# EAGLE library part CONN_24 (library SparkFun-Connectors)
Multi connection point. Often used as Generic Header-pin footprint for 0.1 inch spaced/style header connections On any of the 0.1 inch spaced packages, you can populate with these: Break Away Headers - Straight (PRT-00116) Break Away Male Headers - Right Angle (PRT-00553) Female Headers (PRT-00115) Break Away Headers - Machine Pin (PRT-00117) Break Away Female Headers - Swiss Machine Pin (PRT-00743) For SCREWTERMINALS and SPRING TERMINALS visit here: Screw Terimnals on SparkFun.com (5mm/3.5mm/2.54mm spacing) This device is also useful as a general connection point to wire up your design to another part of your project. Our various solder wires solder well into these plated through hole pads. Hook-Up Wire - Assortment (Stranded, 22 AWG) (PRT-11375) Hook-Up Wire - Assortment (Solid Core, 22 AWG) (PRT-11367) View the entire wire category on our website here Special notes: Molex polarized connector foot print use with SKU : PRT-08231 with associated crimp pins and housings. 1MM SMD Version SKU: PRT-10208 NOTES ON THE VARIANTS LOCK and LOCK_LONGPADS... This footprint was designed to help hold the alignment of a through-hole component (i.e. 6-pin header) while soldering it into place. You may notice that each hole has been shifted either up or down by 0.005 of an inch from it's more standard position (which is a perfectly straight line). This slight alteration caused the pins (the squares in the middle) to touch the edges of the holes. Because they are alternating, it causes a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
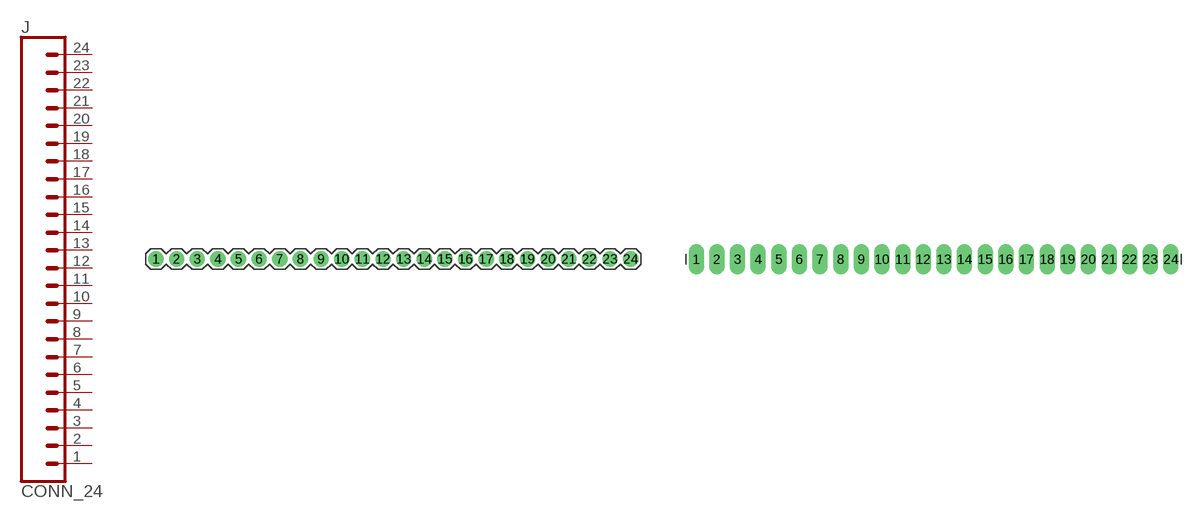
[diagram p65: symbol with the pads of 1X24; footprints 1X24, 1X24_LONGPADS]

Designator prefix J

## CONN_24  [1X24]
1  1  pas
2  2  pas
3  3  pas
4  4  pas
5  5  pas
6  6  pas
7  7  pas
8  8  pas
9  9  pas
10  10  pas
11  11  pas
12  12  pas
13  13  pas
14  14  pas
15  15  pas
16  16  pas
17  17  pas
18  18  pas
19  19  pas
20  20  pas
21  21  pas
22  22  pas
23  23  pas
24  24  pas

## CONN_24LONGPADS  [1X24_LONGPADS]
Pads as for 1X24

## CONN_24LOCK  [1X24_LOCK]
Pads as for 1X24

## Footprint 1X24 (pad centres in mm)
Plated Through Hole -24 Pin Specifications: Pin count:24 Pin pitch:0.1" Example device(s): CONN_24
drill 1.016 pad 1.88: 1 -26.67,0; 2 -24.13,0; 3 -21.59,0; 4 -19.05,0; 5 -16.51,0; 6 -13.97,0; 7 -11.43,0; 8 -8.89,0; 9 -6.35,0; 10 -3.81,0; 11 -1.27,0; 12 1.27,0; 13 3.81,0; 14 6.35,0; 15 8.89,0; 16 11.43,0; 17 13.97,0; 18 16.51,0; 19 19.05,0; 20 21.59,0; 21 24.13,0; 22 26.67,0; 23 29.21,0; 24 31.75,0

## Footprint 1X24_LONGPADS (pad centres in mm)
Plated Through Hole -24 Pin Long Pads Specifications: Pin count:24 Pin pitch:0.1" Example device(s): CONN_24
drill 1.118 pad 1.88 long: 1 -26.67,0; 2 -24.13,0; 3 -21.59,0; 4 -19.05,0; 5 -16.51,0; 6 -13.97,0; 7 -11.43,0; 8 -8.89,0; 9 -6.35,0; 10 -3.81,0; 11 -1.27,0; 12 1.27,0; 13 3.81,0; 14 6.35,0; 15 8.89,0; 16 11.43,0; 17 13.97,0; 18 16.51,0; 19 19.05,0; 20 21.59,0; 21 24.13,0; 22 26.67,0; 23 29.21,0; 24 31.75,0

## Footprint 1X24_LOCK (pad centres in mm)
Plated Through Hole -24 Pin Locking Footprint Holes are offset 0.005" from center, to hold pins in place while soldering. Specifications: Pin count:24 Pin pitch:0.1" Example device(s): CONN_24
drill 1.016 pad 1.88: 1 -26.67,-0.127; 2 -24.13,0.127; 3 -21.59,-0.127; 4 -19.05,0.127; 5 -16.51,-0.127; 6 -13.97,0.127; 7 -11.43,-0.127; 8 -8.89,0.127; 9 -6.35,-0.127; 10 -3.81,0.127; 11 -1.27,-0.127; 12 1.27,0.127; 13 3.81,-0.127; 14 6.35,0.127; 15 8.89,-0.127; 16 11.43,0.127; 17 13.97,-0.127; 18 16.51,0.127; 19 19.05,-0.127; 20 21.59,0.127; 21 24.13,-0.127; 22 26.67,0.127; 23 29.21,-0.127; 24 31.75,0.127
